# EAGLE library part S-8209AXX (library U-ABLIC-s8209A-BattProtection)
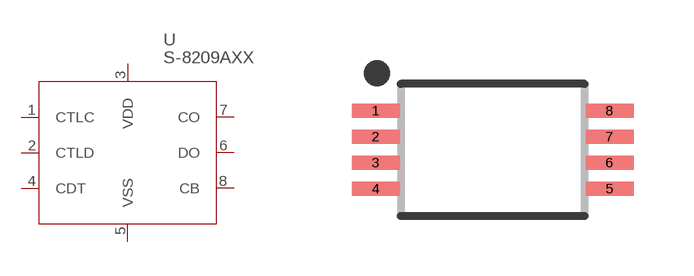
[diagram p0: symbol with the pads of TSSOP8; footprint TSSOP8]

Designator prefix U

## S-8209AXXT  [TSSOP8]
1  CTLC  pas
2  CTLD  in
3  VDD  pwr
4  CDT  pas
5  VSS  pwr
6  DO  oc
7  CO  oc
8  CB  out

## Footprint TSSOP8 (pad centres in mm)
Plastic Small Outline
smd 1.2 x 0.35: 1 -2.925,0.975; 2 -2.925,0.325; 3 -2.925,-0.325; 4 -2.925,-0.975; 5 2.925,-0.975; 6 2.925,-0.325; 7 2.925,0.325; 8 2.925,0.975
